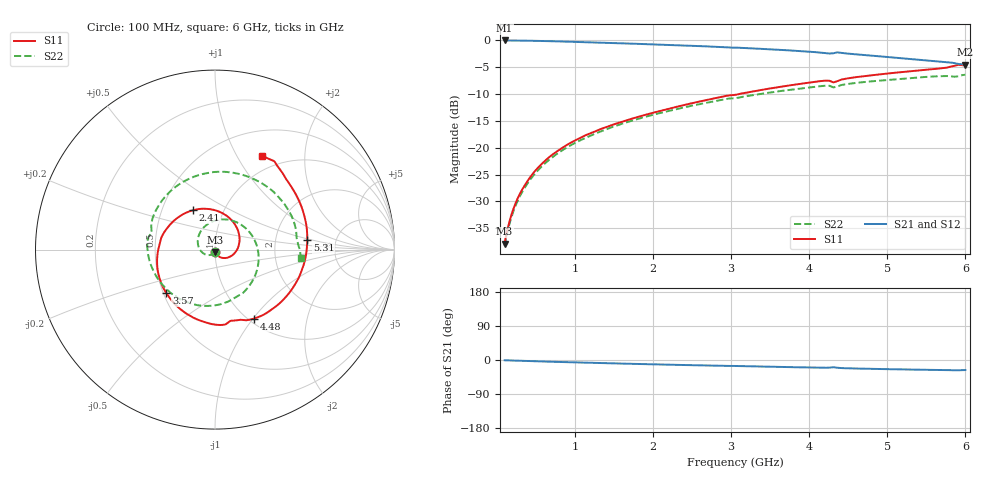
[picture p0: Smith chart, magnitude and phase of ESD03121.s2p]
! Created Thu Jun 14 15:58:37 2018
# hz S ma R 50
! 2 Port Network Data from SP1.SP block
! freq  magS11  angS11  magS21  angS21  magS12  angS12  magS22  angS22
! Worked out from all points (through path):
!   591 points, 100 MHz to 6 GHz, reference 50 ohm
!   highest |S21| = 0.00 dB at 100 MHz (marker M1); lowest = -4.5 dB at 6 GHz (marker M2)
!   group delay of S21, straight-line fit = 12.2 ps
!   lowest |S11| = -37.9 dB at 100 MHz (marker M3), VSWR 1.03, Z = 50.2 - j1.27 ohm
!   |S11| at or under -10 dB: start of sweep to 3.099 GHz
!   |S22| runs from -38.4 to -6.4 dB; largest |S21 - S12| = 0.013
!   S11 on the Smith chart (normalised r, x): 100 MHz: 1.00, -0.03; 2.41 GHz: 0.72, +0.34; 3.57 GHz: 0.52, -0.29; 4.48 GHz: 1.06, -1.01; 5.31 GHz: 3.07, +0.45; 6 GHz: 0.81, +1.28
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1e8  0.01277 -82.1  0.9995 -0.7  0.9998 -0.7  0.01208 -102.4
1.7e8  0.02144 -75.6  0.9988 -1.2  0.999 -1.1  0.0204 -110.9
2.4e8  0.0303 -69.9  0.9977 -1.7  0.9978 -1.6  0.02873 -119.7
4.3e8  0.05341 -54.4  0.9931 -2.9  0.9939 -2.8  0.05069 -143.0
7e8  0.08489 -31.2  0.9834 -4.6  0.9849 -4.4  0.08018 -175.5
1.09e9  0.126 2.3  0.9654 -6.8  0.9686 -6.6  0.1192 139.7
1.62e9  0.1759 49.0  0.939 -9.6  0.9436 -9.4  0.1689 81.7
2.07e9  0.2181 88.9  0.9153 -11.7  0.9207 -11.6  0.2089 34.4
2.41e9  0.2509 119.1  0.8964 -13.3  0.903 -13.1  0.2385 -0.5
2.73e9  0.2827 147.6  0.8776 -14.7  0.8843 -14.6  0.2664 -33.1
3.05e9  0.3107 175.6  0.857 -15.8  0.8647 -15.6  0.289 -65.7
3.32e9  0.3394 -160.2  0.8395 -17.0  0.8482 -17.0  0.3127 -92.8
3.57e9  0.3637 -138.4  0.8212 -18.1  0.8304 -18.0  0.3319 -118.3
4.04e9  0.4075 -98.5  0.782 -20.0  0.7915 -20.0  0.3675 -166.5
4.21e9  0.4216 -85.3  0.7621 -20.4  0.7722 -20.6  0.3786 175.5
4.48e9  0.4413 -60.6  0.7557 -21.8  0.7648 -21.9  0.392 150.3
4.77e9  0.4707 -37.6  0.7241 -23.2  0.7337 -23.4  0.4139 120.5
5.02e9  0.4932 -17.4  0.6998 -24.3  0.7098 -24.5  0.4291 95.1
5.31e9  0.5172 6.0  0.6704 -25.3  0.6813 -25.6  0.4463 65.5
5.68e9  0.5486 37.3  0.6337 -26.3  0.6446 -26.8  0.4648 26.6
5.89e9  0.5881 55.0  0.6077 -27.2  0.618 -27.9  0.4612 5.5
6e9  0.5849 63.2  0.5956 -26.5  0.6055 -27.3  0.4796 -5.9
